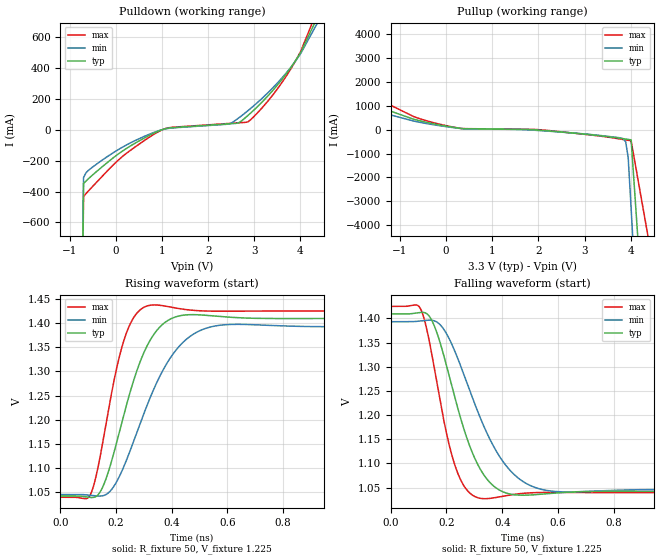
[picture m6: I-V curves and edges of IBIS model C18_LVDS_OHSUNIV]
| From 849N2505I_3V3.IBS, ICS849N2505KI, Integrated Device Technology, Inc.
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[Model]   C18_LVDS_OHSUNIV
Model_type   Output
Polarity   Non-Inverting
|   typ   min   max
C_comp   2pF   1.5pF   2.5pF
Vmeas = 1.225V
Rref = 50
Cref = 0
Vref = 1.225V
|   typ   min   max
[Voltage range]   3.3V   3.135V   3.465V
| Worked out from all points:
|   slope of the pulldown table from 0 to 0.495 V, typ, clamps not added: 5.21 ohm
|   slope of the pullup table from 0 to 0.495 V, typ, clamps not added: 4.43 ohm
|   rising waveform, R_fixture 50, V_fixture 1.225: 20-80 % time 113ps typ, 153ps min, 79.4ps max; typ from 1.04 V to 1.41 V
|   falling waveform, R_fixture 50, V_fixture 1.225: 20-80 % time 113ps typ, 153ps min, 79.4ps max; typ from 1.41 V to 1.04 V
[Pulldown]
|Voltage   I (typ)   I (min)   I (max)
-3.3V     -101A      -86.78A    -125A
-1.22V    -14.69A    -15.06A    -14.32A
-700mV    -348.2mA   -309.7mA   -433mA
-537mV    -301.6mA   -249.3mA   -378mA
165.2mV   -133.8mA   -109.3mA   -168mA
1.029V    2.521mA    2.336mA    2.643mA
2.434V    37.5mA     35.9mA     40.12mA
2.866V    93.09mA    124.1mA    51.39mA
3.46V     274.6mA    289.3mA    247.9mA
4.01V     502.2mA    495.8mA    509.9mA
4.528V    829.8mA    777.5mA    894.2mA
6.6V      11.43A     11.38A     11.74A
[Pullup]
|Voltage   I (typ)   I (min)   I (max)
-3.3V     11.48A     10.42A     13.36A
-2.78V    7.713A     7.303A     8.515A
-2.26V    3.971A     4.203A     3.697A
-1.74V    1.318A     1.228A     1.814A
-1.22V    791.2mA    629mA      1.045A
327.2mV   52.08mA    48.11mA    53.39mA
3.838V    -377.5mA   -379mA     -410.5mA
3.892V    -391.9mA   -506.1mA   -427.3mA
3.946V    -406.8mA   -1.162A    -444.5mA
4.01V     -426mA     -3.307A    -465mA
4.528V    -15.08A    -21.05A    -6.139A
6.6V      -100.9A    -92.43A    -116A
[Ramp]
|   typ   min   max
dV/dt_r   0.302/0.176n   0.284/0.236n   0.32/0.124n
dV/dt_f   0.302/0.176n   0.284/0.236n   0.32/0.124n
R_load =   50.0000
[Rising Waveform]
R_fixture = 50
V_fixture = 1.225   |Vcc_typ
V_fixture_min = 1.2  |Vcc_min
V_fixture_max = 1.23 |Vcc_max
C_fixture = 0.0p
| Time   typ   min   max
0s        1.042V     1.045V     1.04V
110.1ps   1.039V     1.043V     1.048V
156.4ps   1.067V     1.043V     1.167V
221.5ps   1.196V     1.094V     1.351V
257.8ps   1.271V     1.147V     1.406V
300.3ps   1.339V     1.213V     1.433V
349.1ps   1.387V     1.28V      1.437V
405.4ps   1.411V     1.336V     1.432V
524.3ps   1.416V     1.389V     1.425V
1.25ns    1.41V      1.392V     1.425V
[Falling Waveform]
R_fixture = 50
V_fixture = 1.225   |Vcc_typ
V_fixture_min = 1.2  |Vcc_min
V_fixture_max = 1.23 |Vcc_max
C_fixture = 0.0p
| Time   typ   min   max
0s        1.409V     1.393V     1.425V
110.1ps   1.413V     1.395V     1.416V
156.4ps   1.385V     1.395V     1.298V
221.5ps   1.256V     1.344V     1.113V
257.8ps   1.18V      1.291V     1.059V
300.3ps   1.112V     1.225V     1.032V
349.1ps   1.065V     1.158V     1.027V
405.4ps   1.041V     1.102V     1.032V
524.3ps   1.036V     1.049V     1.04V
1.25ns    1.042V     1.046V     1.039V
